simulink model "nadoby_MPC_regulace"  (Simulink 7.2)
settings: Solver=ode15s  StartTime=0.0  StopTime=900  RelTol=1e-3
undefined symbols (not defined in the file or in its folder): Humusoft, MF624, to, V
libraries: rtlib x3, simulink x2, mpclib x1

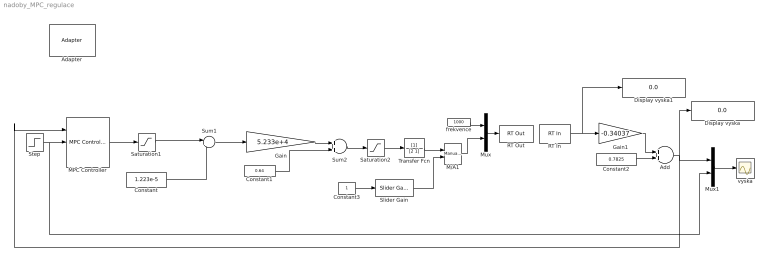
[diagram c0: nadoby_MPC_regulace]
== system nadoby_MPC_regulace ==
  Adapter : rtlib/Adapter  SystemSampleTime=-1  DriverName=Humusoft/MF624  DriverAddress=4294967295  DriverOptions=1
  Add : Sum  OutDataType=sfix(16)  OutScaling=2^-10
  Constant : Constant  Value=1.223e-5  OutDataType=fixdt(1, 16)  OutScaling=2^0
  Constant1 : Constant  Value=0.64  OutDataType=fixdt(1, 16)  OutScaling=2^0
  Constant2 : Constant  Value=0.7825  OutDataType=sfix(16)  OutScaling=2^0
  Constant3 : Constant  OutDataType=fixdt(1, 16)  OutScaling=2^0
  Display vyska : Display
  Display vyska1 : Display
  Gain : Gain  Gain=5.233e+4  ParameterDataType=sfix(16)  ParameterScaling=2^0  OutDataType=sfix(16)  OutScaling=2^0
  Gain1 : Gain  Gain=-0.34037  ParameterDataType=sfix(16)  ParameterScaling=2^0  OutDataType=sfix(16)  OutScaling=2^0
  M/A1 : simulink/Signal Routing/Manual Switch  SystemSampleTime=-1  sw=0  action=0  varsize=off
  MPC Controller : mpclib/MPC Controller  SystemSampleTime=-1  mpcobj=mpc_controller  n_mv=0  x0=[]  ref_from_ws=off  ref_signal_name=[]  ref_preview=on  md_from_ws=off  md_signal_name=[]  md_preview=on  from_project=off  md_inport=on  mv_inport=off  lims_inport=off  switch_inport=off  enable_value=0  project_file=MPCtask.mat  is_multiple=0
  Mux : Mux  Inputs=2
  Mux1 : Mux  Inputs=2
  RT In : rtlib/RT In  SampleTime=0.1  Adapter=Adapter  IOClass=Analog Input  Channels=1  SLDataType=double  MaxMissedTicks=inf  ShowMissedTicks=off  YieldWhenWaiting=on  AIORange=-10 to 10 V  AIOUnits=Volts  DIOMode=Bit  CIReset=never  CIEdge=rising  CIGate=none  EIQuadrature=quadruple  EIIndexPulse=reset  EIFilterFrequency=Inf  OIOParameters=[]
  RT Out : rtlib/RT Out  SampleTime=0.1  Adapter=Adapter  IOClass=Other Output  Channels=[1 2]  InitialValue=[]  FinalValue=[]  MaxMissedTicks=inf  ShowMissedTicks=off  YieldWhenWaiting=on  AIORange=-10 to 10 V  AIOUnits=Volts  DIOMode=Bit  OIOParameters=[]
  Saturation1 : Saturate  UpperLimit=1.9109e-5  LowerLimit=0  ZeroCross=off  OutDataType=fixdt(1, 16)  OutScaling=2^0
  Saturation2 : Saturate  UpperLimit=1  LowerLimit=0.37  ZeroCross=off  OutDataType=fixdt(1, 16)  OutScaling=2^0
  Slider Gain : simulink/Math Operations/Slider Gain  SystemSampleTime=-1  low=0  gain=0  high=1
  Step : Step  Time=700  Before=0.35  After=0.3  SampleTime=0
  Sum1 : Sum  Inputs=|+-  OutDataType=fixdt(1, 16)  OutScaling=2^0
  Sum2 : Sum  OutDataType=fixdt(1, 16)  OutScaling=2^0
  Transfer Fcn : TransferFcn  Denominator=[2 1]
  frekvence : Constant  Value=1000  OutDataType=fixdt(1, 16)  OutScaling=2^0
  vyska : Scope
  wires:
  Sum1/1 -> Gain/1
  MPC Controller/1 -> Saturation1/1
  frekvence/1 -> Mux/1
  Gain1/1 -> Add/1
  Constant2/1 -> Add/2
  RT In/1 -> Gain1/1, Display vyska1/1
  Step/1 -> MPC Controller/2, Mux1/2
  Gain/1 -> Sum2/1
  Mux/1 -> RT Out/1
  Constant3/1 -> Slider Gain/1
  Constant1/1 -> Sum2/2
  Saturation2/1 -> Transfer Fcn/1
  Saturation1/1 -> Sum1/1
  Constant/1 -> Sum1/2
  Add/1 -> MPC Controller/1, Mux1/1, Display vyska/1
  Mux1/1 -> vyska/1
  Sum2/1 -> Saturation2/1
  Transfer Fcn/1 -> M/A1/1
  M/A1/1 -> Mux/2
  Slider Gain/1 -> M/A1/2
